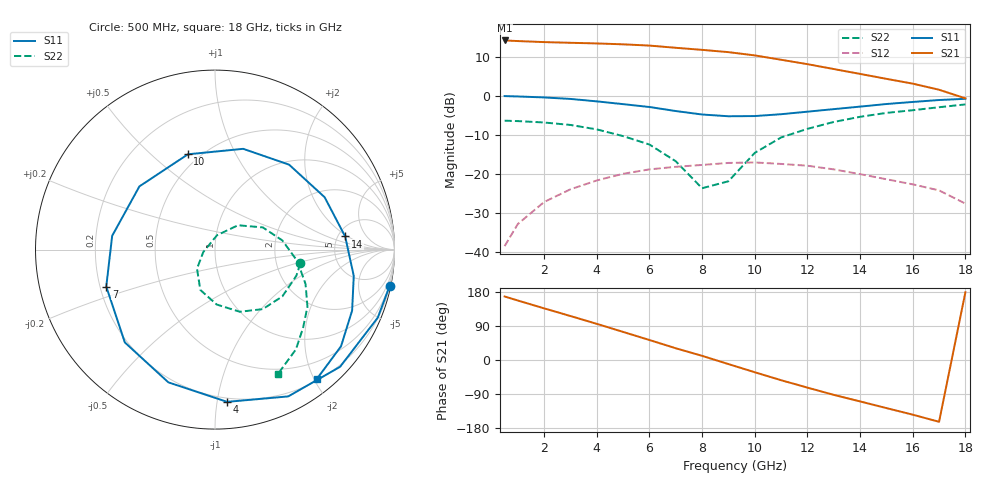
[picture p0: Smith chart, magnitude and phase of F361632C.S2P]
!ATF-36163
!2V 20mA
! last updated 11-10-95
# ghz s ma r 50
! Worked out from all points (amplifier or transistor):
!   19 points, 500 MHz to 18 GHz, reference 50 ohm
!   highest |S21| = 14.2 dB at 500 MHz (marker M1)
!   |S21| within 3 dB of that: start of sweep to 9.017 GHz
!   unconditionally stable (mu >= 1): 10.22 GHz to end of sweep
!   at 3 GHz: K = 0.36, MSG = 18.7 dB, |S12| = -23.9 dB
!   at 9 GHz: K = 0.93, MSG = 14.2 dB, |S12| = -17.1 dB
!   at 18 GHz: K = 1.42, MAG = 9.6 dB, |S12| = -27.5 dB
!   lowest NFmin = 0.52 dB at 2 GHz
!   S11 on the Smith chart (normalised r, x): 500 MHz: 0.29, -9.72; 4 GHz: 0.17, -1.07; 7 GHz: 0.23, -0.16; 10 GHz: 0.43, +0.66; 14 GHz: 5.80, +1.81; 18 GHz: 0.22, -2.03
0.5  0.994 -11.7  5.108 167.7  0.012 79.2  0.482 -9.1
1  0.983 -22.7  5.019 157.0  0.023 71.5  0.476 -17.9
2  0.955 -43.1  4.867 136.3  0.044 56.0  0.457 -34.8
3  0.914 -63.5  4.768 116.0  0.064 40.7  0.425 -51.2
4  0.851 -85.4  4.68 95.4  0.083 24.4  0.373 -68.2
5  0.784 -109.3  4.557 74.1  0.101 7.2  0.306 -88.3
6  0.721 -134.2  4.393 52.7  0.115 -9.5  0.239 -110.0
7  0.64 -161.2  4.116 31.0  0.124 -26.9  0.146 -133.3
8  0.578 172.4  3.873 11.0  0.131 -39.9  0.066 -169.0
9  0.549 140.1  3.622 -10.8  0.139 -54.6  0.081 81.8
10  0.552 105.9  3.29 -32.3  0.141 -69.7  0.187 46.5
11  0.583 74.4  2.894 -53.3  0.135 -84.2  0.294 24.8
12  0.628 48.9  2.544 -72.9  0.128 -96.7  0.379 7.7
13  0.677 25.5  2.203 -92.0  0.115 -109.0  0.464 -8.1
14  0.729 5.7  1.909 -109.3  0.1 -117.8  0.54 -20.9
15  0.787 -10.8  1.651 -126.9  0.086 -126.2  0.606 -31.8
16  0.836 -23.9  1.433 -144.3  0.074 -132.0  0.656 -41.6
17  0.885 -37.5  1.198 -163.1  0.062 -139.9  0.716 -51.0
18  0.918 -51.9  0.93 178.8  0.042 -146.8  0.778 -63.4
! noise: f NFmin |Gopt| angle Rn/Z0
2  0.52  0.826  28.08  0.393
3  0.57  0.746  41.9  0.323
5  0.66  0.591  72.65  0.2
7  0.76  0.46  105.7  0.115
9  0.88  0.299  140.4  0.077
10  0.94  0.199  174.5  0.079
12  1.09  0.201  -79.72  0.149
14  1.28  0.38  -12.57  0.356
16  1.52  0.613  20.98  0.658
18  1.85  0.758  52.86  1.215
